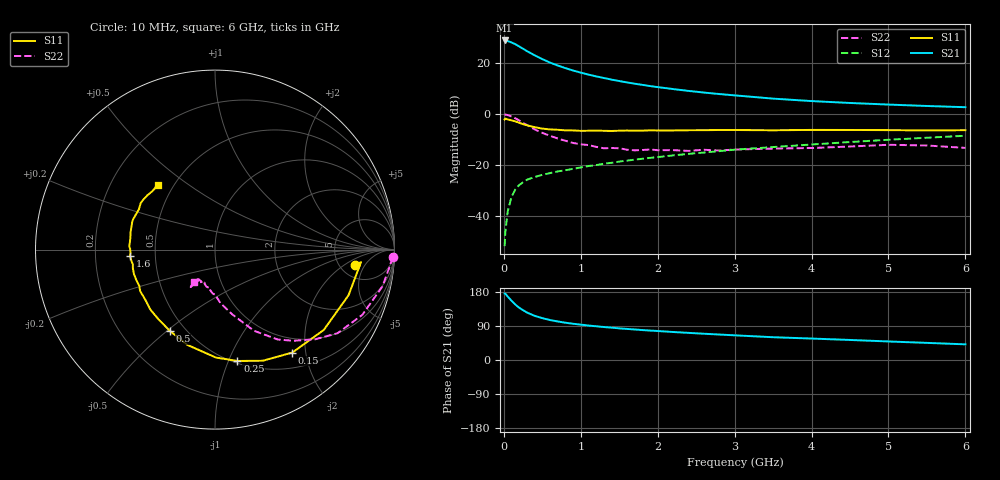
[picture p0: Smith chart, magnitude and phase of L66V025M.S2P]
!  INFINEON TECHNOLOGIES Small Signal Semiconductors
! BFR380L3 , Si-NPN RF-Transistor in TSLP-3-1
!  Vce=6 V,  Ic=25 mA
! Common Emitter S-Parameters:  07. March 2005
#  GHz  S  MA  R  50
! f  S11  S21  S12  S22
! GHz  Mag  Ang  Mag  Ang  Mag  Ang  Mag  Ang
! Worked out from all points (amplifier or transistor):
!   36 points, 10 MHz to 6 GHz, reference 50 ohm
!   highest |S21| = 29.0 dB at 10 MHz (marker M1)
!   |S21| within 3 dB of that: start of sweep to 235.4 MHz
!   unconditionally stable (mu >= 1): 2.266 GHz to 4.72 GHz
!   at 250 MHz: K = 0.32, MSG = 26.3 dB, |S12| = -26.8 dB
!   at 1.4 GHz: K = 0.91, MSG = 16.4 dB, |S12| = -19.2 dB
!   at 6 GHz: K = 0.97, MSG = 5.6 dB, |S12| = -8.5 dB
!   S11 on the Smith chart (normalised r, x): 10 MHz: 6.97, -3.11; 150 MHz: 0.74, -1.76; 250 MHz: 0.52, -1.08; 500 MHz: 0.41, -0.51; 1.6 GHz: 0.36, -0.03; 6 GHz: 0.41, +0.39
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0.01  0.7868 -6.2  28.25 175.4  0.0025 67.4  0.9898 -2.4
0.02  0.8166 -4.9  28.14 175.0  0.0048 78.1  0.9794 -5.1
0.05  0.7862 -18.9  27.51 167.5  0.012 79.8  0.9559 -12.3
0.1  0.7536 -36.4  25.81 156.3  0.0235 72.1  0.8977 -23.9
0.15  0.7174 -53.1  23.8 146.2  0.0329 65.9  0.8267 -34.3
0.2  0.6742 -66.7  21.51 137.9  0.0401 62.1  0.7496 -41.8
0.25  0.633 -78.6  19.41 131.3  0.0455 57.4  0.6702 -49.3
0.3  0.6015 -89.5  17.45 125.4  0.0509 55.4  0.6108 -55.1
0.4  0.5527 -106.3  14.41 116.6  0.0576 52.3  0.5013 -64.4
0.5  0.518 -119.1  12.12 110.5  0.0636 51.5  0.4262 -69.7
0.6  0.4993 -129.4  10.36 105.5  0.0688 51.5  0.3734 -75.1
0.7  0.4913 -137.1  9.076 101.7  0.0743 52.5  0.3308 -79.7
0.9  0.4768 -151.0  7.218 95.7  0.0834 54.2  0.2696 -87.5
1.1  0.4701 -159.3  6.005 90.9  0.0947 56.2  0.2455 -93.0
1.4  0.4651 -169.7  4.784 85.4  0.1098 58.0  0.2148 -99.4
1.6  0.4743 -176.0  4.214 82.0  0.1211 59.0  0.1989 -107.1
2.2  0.4763 171.8  3.114 73.9  0.1536 61.1  0.1948 -112.4
2.8  0.4866 161.4  2.486 67.2  0.1864 62.1  0.1916 -120.4
3.5  0.4798 152.0  2.019 60.1  0.2241 61.3  0.2093 -121.3
4.5  0.4869 145.2  1.657 52.9  0.2819 60.8  0.2298 -122.5
5.5  0.4771 137.0  1.445 45.2  0.3425 58.0  0.2407 -122.9
6  0.4819 131.4  1.368 41.3  0.3746 56.2  0.2159 -123.6
